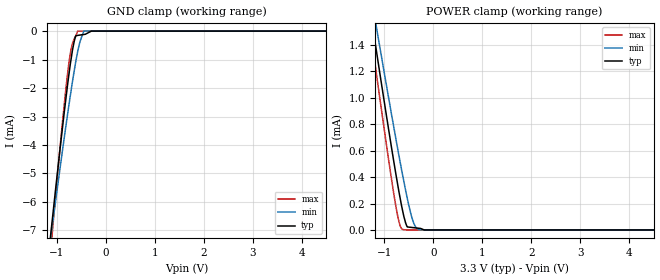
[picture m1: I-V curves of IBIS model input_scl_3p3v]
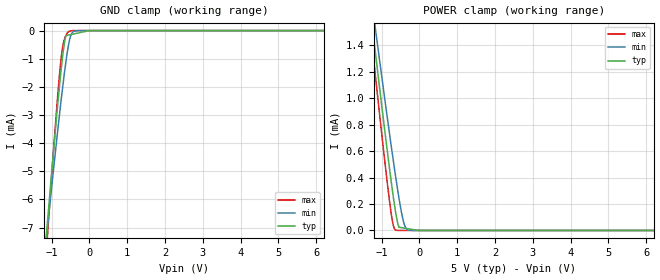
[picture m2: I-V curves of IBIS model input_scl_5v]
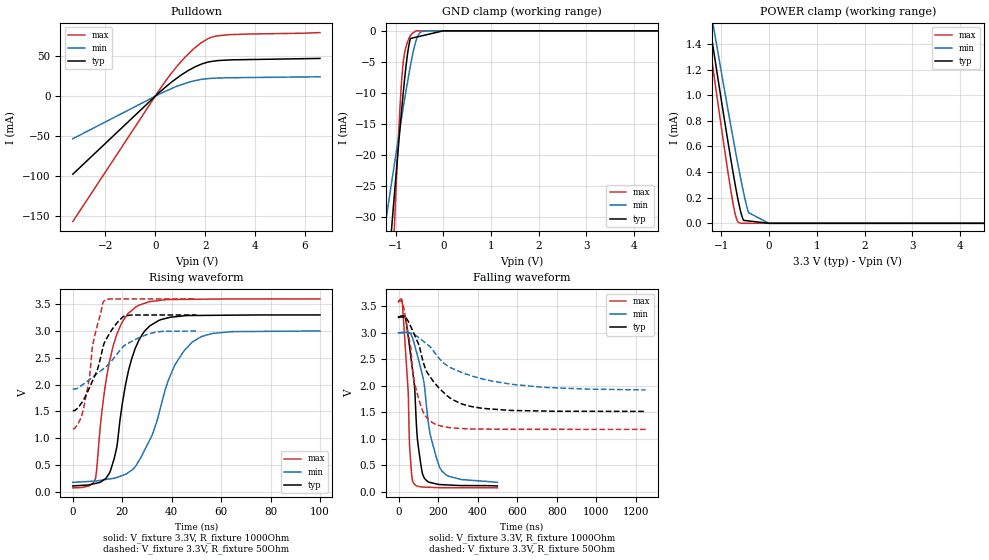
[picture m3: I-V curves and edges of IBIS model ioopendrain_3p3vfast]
|Texas Instruments Incorporated
| 10-bit, Quad, Digital-to-Analog Converter with I2C interface
| Marketing part#   Digital Voltage Range   Package-type   #pins
| DAC6574IDGS   2.7 to 5.5V   MSOP   10
| DAC6574IDGSG4   2.7 to 5.5V   MSOP   10
| DAC6574IDGSR   2.7 to 5.5V   MSOP   10
| DAC6574IDGSRG4   2.7 to 5.5V   MSOP   10
[IBIS Ver]   3.2
[File name]   dac6574.ibs
|SIMDE Ver   V2.1 - 201006 - RHL4 - Build 390
[File Rev]   1.0
[Date]   10/29/2010
[Source]
| Texas Instruments Incorporated.
| Analog-eLab Design Center, HPA
| 12500 TI Blvd
| Dallas, TX -75243
| e-mail: elab_ibis@list.ti.com
| -Model generated from simulations in SPECTRE
[Notes]   Revision History:
| Rev 1.0: 10/29/2010
| - Initial version of the model
| - Model generated from simulations in SPECTRE
| - Model matched to SPICE simulation
| - C_comp although listed in numerical order of value are
|   obtained from varying PVT conditions. For PVT conditions for
|   each specific value refer the buffer description under
|   respective [Model]. IBIS model user is responsible for using
|   appropriate C_comp to simulate for Signal Integrity.
| - Models A0 and A1 same as that of SCL
[Disclaimer]
| This model is designed as an aid for customers of Texas Instruments.
| TI and its licensors and suppliers make no warranties, either expressed
| or implied, with respect to this  model, including the warranties of
| merchantability or fitness for a particular purpose. The model is
| provided solely on an "as is" basis. The entire risk as to its quality
| and performance is with the customer.
[Copyright]
 (C) Copyright 2010 Texas Instruments Incorporated.All rights reserved.
|   DAC6574
[Component]   DAC6574
[Manufacturer]   TI
[Package]   |10 MSOP -  DGS package
|   typ   min   max
R_pkg   0.042886   0.04198   0.04381
L_pkg   1.316828nH   1.29136nH   1.34345nH
C_pkg   0.22412pF   0.20777pF   0.24149pF
[Pin]  signal_name   model_name   R_pin   L_pin   C_pin
1   VOUTA   TERM   0.04361   1.33655nH  0.21059pF
2   VOUTB   TERM   0.04270   1.30706nH  0.24149pF
3   GND   GND   0.02248   1.15319nH  0.25862pF
4   VOUTC   TERM   0.04237   1.29999nH  0.23814pF
5   VOUTD   TERM   0.04361   1.33922nH  0.20815pF
6   SCL   INPUT_SCL   0.04381   1.34245nH  0.20902pF
7   SDA   IOOPENDRAIN   0.04198   1.29136nH  0.23809pF
8   VDD   POWER   0.02243   1.14887nH  0.25838pF
9   A0   INPUT_SCL   0.04241   1.30080nH  0.23971pF
10   A1   INPUT_SCL   0.04260   1.31619nH  0.20777pF
|   Model Selectors
[Model Selector] INPUT_SCL
input_scl_3p3v 3.3V digital input
input_scl_5v   5.0V digital input
[Model Selector] IOOPENDRAIN
ioopendrain_3p3vfast 3.3V digital ioopendrain in fast mode (3.4MHz,Rload=1k)
ioopendrain_3p3vstd  3.3V digital ioopendrain in std mode (100KHz,Rload=10k)
ioopendrain_5v_fast  5V   digital ioopendrain in fast mode (3.4MHz,Rload=1k)
ioopendrain_5v_std   5V   digital ioopendrain in std mode (100KHz,Rload=10k)
[Model Selector] TERM
TERM_3p3  3.3V nominal termination
TERM_5   5.0V nominal termination
[Model] TERM_3p3
Model_type Terminator
C_comp   1.0e-20F  1.0e-20F  1.0e-20F
|   typ   min   max
[Voltage Range]   3.3V   3.0V   3.6V
[POWER Clamp Reference]   3.3V   3.0V   3.6V
[GND Clamp Reference]   0V   0V   0V
|Ambient Temperature   25   105   -40
|Junction Temperature
[Temperature Range]   25   105   -40
[Model] TERM_5
Model_type Terminator
C_comp   1.0e-20F  1.0e-20F  1.0e-20F
|   typ   min   max
[Voltage Range]   5.0V   4.5V   5.5V
[POWER Clamp Reference]   5.0V   4.5V   5.5V
[GND Clamp Reference]   0V   0V   0V
|Ambient Temperature   25   105   -40
|Junction Temperature
[Temperature Range]   25   105   -40
| Models and submodels in the file (8): input_scl_3p3v (Input), input_scl_5v (Input), ioopendrain_3p3vfast (I/O_open_drain), ioopendrain_3p3vstd (I/O_open_drain), ioopendrain_5v_fast (I/O_open_drain), ioopendrain_5v_std (I/O_open_drain), TERM_3p3 (Terminator), TERM_5 (Terminator)
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|   input_scl_3p3v Model
[Model]   input_scl_3p3v
Model_type   Input
Vinl = 0.99
Vinh = 2.31
|   typ   min   max
|   (nom PVT)   (Fast PVT)   (slow PVT)
|Average
C_comp   4.196e-12   4.137e-12   4.262e-12
| Where nom  PVT is Nominal Process, 3.3V, 25C
|   Fast PVT is Strong Process,  3.6V, -40C
|   Slow PVT is Weak Process,   3V, 105C
[Model spec]
|   typ   min   max
Vinl   0.99   0.9   1.08
Vinh   2.31   2.1   2.52
[Voltage Range]   3.3   3   3.6
|Ambient Temperature   25   105   -40
|Junction Temperature
[Temperature Range]   25   105   -40
[Power Clamp Reference]   3.3   3   3.6
[GND Clamp Reference]   0   0   0
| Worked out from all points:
|   GND clamp passes 1 mA (typ) near -0.71 V on its own axis
|   POWER clamp passes 1 mA (typ) near -1.02 V on its own axis
[GND Clamp]
|   Voltage   I(typ)   I(min)   I(max)
-3.3V     -43.31mA   -36.41mA   -55.69mA
-1.142V   -7.355mA   -7.431mA   -8.009mA
-1.083V   -6.42mA    -6.667mA   -6.829mA
-895.2mV  -3.502mA   -4.282mA   -3.319mA
-758.4mV  -1.548mA   -2.621mA   -1.146mA
-704.4mV  -898.6uA   -2.005mA   -572.4uA
-650.1mV  -375.1uA   -1.416mA   -283.2uA
-613.8mV  -161.6uA   -1.05mA    -162.8uA
-578.4mV  -152.3uA   -729.3uA   0A
-453mV    -119.3uA   0A         0A
-297mV    0A         0A         0A
6.6V      0A         0A         0A
[POWER Clamp]
|   Voltage   I(typ)   I(min)   I(max)
-3.3V     6.651mA    6.278mA    7.033mA
-1.313V   1.712mA    1.855mA    1.577mA
-1.247V   1.552mA    1.712mA    1.401mA
-1.154V   1.327mA    1.51mA     1.152mA
-873.6mV  662.5uA    910uA      425.5uA
-762mV    411.2uA    678.4uA    166.8uA
-690mV    259.4uA    532.3uA    42.61uA
-621.6mV  131.7uA    399.4uA    2.885uA
-534.6mV  22.99uA    239.9uA    49.29nA
-411mV    17.67uA    60.06uA    37.86nA
-261mV    11.22uA    1.335uA    24nA
6.6V      0A         0A         0A
|   input_scl_5v Model
[Model]   input_scl_5v
Model_type   Input
Vinl = 1.5
Vinh = 3.5
|   typ   min   max
|   (nom PVT)   (Fast PVT)   (slow PVT)
|Average
C_comp   4.159e-12   4.107e-12   4.214e-12
| Where nom  PVT is Nominal Process, 5V, 25C
|   Fast PVT is Strong Process,  5.5V, -40C
|   Slow PVT is Weak Process,   4.5V, 105C
[Model spec]
|   typ   min   max
Vinl   1.5   1.35   1.65
Vinh   3.5   3.15   3.85
[Voltage Range]   5   4.5   5.5
|Ambient Temperature   25   105   -40
|Junction Temperature
[Temperature Range]   25   105   -40
[Power Clamp Reference]   5   4.5   5.5
[GND Clamp Reference]   0   0   0
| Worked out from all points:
|   GND clamp passes 1 mA (typ) near -0.72 V on its own axis
|   POWER clamp passes 1 mA (typ) near -1.02 V on its own axis
[GND Clamp]
|   Voltage   I(typ)   I(min)   I(max)
-5V       -71.99mA   -59.56mA   -93.94mA
-1.153V   -7.505mA   -7.546mA   -8.189mA
-1.089V   -6.495mA   -6.736mA   -6.914mA
-875mV    -3.167mA   -4.015mA   -2.935mA
-798mV    -2.065mA   -3.081mA   -1.679mA
-737.5mV  -1.269mA   -2.359mA   -866.6uA
-688mV    -709.2uA   -1.807mA   -445.5uA
-620mV    -180.1uA   -1.101mA   -175.8uA
-528.5mV  -153.4uA   -353.8uA   -20.04uA
-459.5mV  -133.2uA   -81.14uA   -4.502uA
-288.5mV  -83.23uA   0A         0A
10V       0A         0A         0A
[POWER Clamp]
|   Voltage   I(typ)   I(min)   I(max)
-5V       10.91mA    10.1mA     11.74mA
-1.34V    1.773mA    1.91mA     1.644mA
-1.265V   1.591mA    1.746mA    1.442mA
-1.222V   1.485mA    1.652mA    1.325mA
-1.155V   1.324mA    1.508mA    1.149mA
-765mV    412.6uA    680.4uA    167.9uA
-688mV    250.4uA    525.7uA    36.76uA
-627.5mV  136.3uA    406uA      2.254uA
-540mV    24.35uA    244.8uA    0A
-450.5mV  20.14uA    104uA      0A
-306.5mV  13.37uA    3.888uA    0A
10V       0A         0A         0A
|   ioopendrain_3p3vfast Model
[Model]   ioopendrain_3p3vfast
Model_type   I/O_open_drain
Polarity   Non-Inverting
Enable   Active-Low
Vinl = 0.99
Vinh = 2.31
Vmeas = 1.65
Vref = 3.3
Cref = 15pF
Rref = 1000
|   typ   min   max
|   (nom PVT)   (Fast PVT)   (slow PVT)
|Average
C_comp   5.117e-12   5.087e-12   5.165e-12
|ON state : BUFFER OUTPUT TURNED LOW
|C_comp   8.694e-11   4.037e-11   1.679e-10
|OFF state: BUFFER in HIGH IMPEDANCE
|C_comp   5.117e-12   5.087e-12   5.165e-12
| Where nom  PVT is Nominal Process, 3.3V, 25C
|   Fast PVT is Strong Process,  3.6V, -40C
|   Slow PVT is Weak Process,   3V, 105C
[Model spec]
|   typ   min   max
Vinl   0.99   0.9   1.08
Vinh   2.31   2.1   2.52
[Voltage Range]   3.3   3   3.6
|Ambient Temperature   25   105   -40
|Junction Temperature
[Temperature Range]   25   105   -40
[Pullup Reference]   3.3   3   3.6
[Pulldown Reference]   0   0   0
[Power Clamp Reference]   3.3   3   3.6
[GND Clamp Reference]   0   0   0
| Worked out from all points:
|   slope of the pulldown table from 0 to 0.495 V, typ, clamps not added: 36.2 ohm
|   GND clamp passes 1 mA (typ) near -0.56 V on its own axis
|   POWER clamp passes 1 mA (typ) near -1.02 V on its own axis
|   falling waveform, V_fixture 3.3V, R_fixture 1000Ohm: 20-80 % time 45.6ns typ, 79.6ns min, 26.2ns max; typ from 3.3 V to 0.11 V
|   rising waveform, V_fixture 3.3V, R_fixture 1000Ohm: 20-80 % time 7.76ns typ, 13.6ns min, 7.19ns max; typ from 0.11 V to 3.3 V
|   falling waveform, V_fixture 3.3V, R_fixture 50Ohm: 20-80 % time 145ns typ, 273ns min, 66.4ns max; typ from 3.3 V to 1.52 V
|   rising waveform, V_fixture 3.3V, R_fixture 50Ohm: 20-80 % time 8.67ns typ, 15ns min, 5.15ns max; typ from 1.52 V to 3.3 V
[Pulldown]
|   Voltage   I(typ)   I(min)   I(max)
-3.3V     -97.88mA   -53.33mA   -157.4mA
318mV     9.006mA    5.005mA    14.9mA
876mV     22.96mA    12.66mA    37.86mA
1.204V    29.99mA    16.21mA    49.42mA
1.52V     35.68mA    19.08mA    59.08mA
1.823V    40.01mA    21.17mA    66.75mA
2.262V    43.76mA    22.62mA    74.29mA
2.942V    45.57mA    23.31mA    77.37mA
6.6V      47.55mA    24.48mA    80.03mA
[GND Clamp]
|   Voltage   I(typ)   I(min)   I(max)
-3.3V     -246.7mA   -140.1mA   -463.1mA
-1.269V   -49.35mA   -33.72mA   -76.76mA
-1.208V   -43.43mA   -30.6mA    -65.2mA
-1.072V   -30.43mA   -23.65mA   -39.58mA
-1.047V   -28.13mA   -22.41mA   -35.08mA
-1.021V   -25.74mA   -21.13mA   -30.4mA
-913.2mV  -15.96mA   -15.79mA   -12.69mA
-837.6mV  -9.656mA   -12.16mA   -4.795mA
-706.2mV  -1.692mA   -6.233mA   -973.9uA
-574.8mV  -1.018mA   -1.632mA   0A
-330mV    -584.6uA   0A         0A
6.6V      0A         0A         0A
[POWER Clamp]
|   Voltage   I(typ)   I(min)   I(max)
-3.3V     6.651mA    6.278mA    7.033mA
-1.313V   1.712mA    1.855mA    1.577mA
-1.247V   1.552mA    1.712mA    1.401mA
-1.154V   1.327mA    1.51mA     1.152mA
-873.6mV  662.5uA    910uA      425.5uA
-762mV    411.2uA    678.4uA    166.8uA
-690mV    259.4uA    532.3uA    42.61uA
-621.6mV  131.7uA    399.4uA    2.885uA
-534.6mV  22.99uA    239.9uA    49.42nA
-432mV    18.58uA    83.42uA    39.92nA
-3mV      129nA      0A         203pA
6.6V      0A         0A         0A
[Ramp]
R_load = 1000
|   typ   min   max
dV/dt_r   1.91424/7.70728e-09   1.69415/1.34473e-08   2.11566/7.16003e-09
dV/dt_f   1.91424/4.55019e-08   1.69404/7.9201e-08   2.11566/2.60725e-08
[Falling Waveform]
V_fixture = 3.3V
V_fixture_min = 3V
V_fixture_max = 3.6V
R_fixture = 1000Ohm
|   Time   V(typ)   V(min)   V(max)
0s        3.3V       3V         3.6V
19.83ns   3.32V      3.011V     3.534V
48.96ns   2.932V     3.008V     1.882V
56.61ns   2.716V     2.997V     831.8mV
75.31ns   2.168V     2.852V     166.8mV
95.56ns   991.5mV    2.573V     107.5mV
131ns     252.5mV    1.998V     87.54mV
162.2ns   173.2mV    1.047V     83.35mV
220.1ns   133.8mV    387.2mV    76.47mV
500ns     109.6mV    176.6mV    73.9mV
[Rising Waveform]
V_fixture = 3.3V
V_fixture_min = 3V
V_fixture_max = 3.6V
R_fixture = 1000Ohm
|   Time   V(typ)   V(min)   V(max)
0s        109.6mV    176.4mV    73.9mV
9.116ns   156.6mV    200mV      240.7mV
11.87ns   201.6mV    219.2mV    1.536V
14.9ns    355.1mV    240.6mV    2.445V
17.74ns   819.6mV    265.9mV    2.93V
19.48ns   1.466V     295.5mV    3.122V
25.78ns   2.731V     504mV      3.458V
41.26ns   3.266V     2.364V     3.589V
48.31ns   3.29V      2.794V     3.592V
100ns     3.3V       3V         3.6V
[Falling Waveform]
V_fixture = 3.3V
V_fixture_min = 3V
V_fixture_max = 3.6V
R_fixture = 50Ohm
|   Time   V(typ)   V(min)   V(max)
0s        3.3V       3V         3.6V
25.08ns   3.299V     3V         3.498V
62.23ns   3.116V     2.994V     2.709V
77.05ns   2.994V     2.976V     2.129V
101.7ns   2.785V     2.912V     1.758V
137.1ns   2.313V     2.806V     1.425V
175.3ns   2.09V      2.665V     1.296V
274.4ns   1.738V     2.324V     1.206V
424.7ns   1.575V     2.131V     1.183V
1.25us    1.517V     1.923V     1.178V
[Rising Waveform]
V_fixture = 3.3V
V_fixture_min = 3V
V_fixture_max = 3.6V
R_fixture = 50Ohm
|   Time   V(typ)   V(min)   V(max)
0s        1.517V     1.917V     1.178V
2.198ns   1.577V     1.94V      1.275V
4.203ns   1.705V     2.006V     1.526V
6.676ns   1.936V     2.092V     2.115V
8.195ns   2.092V     2.146V     2.771V
10.05ns   2.292V     2.213V     3.13V
12.56ns   2.756V     2.302V     3.559V
20.54ns   3.273V     2.716V     3.599V
33.35ns   3.299V     2.978V     3.599V
50ns      3.3V       3V         3.6V
